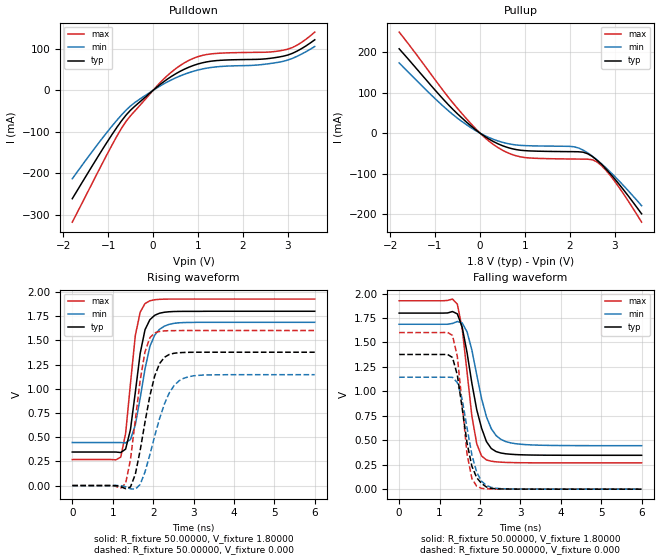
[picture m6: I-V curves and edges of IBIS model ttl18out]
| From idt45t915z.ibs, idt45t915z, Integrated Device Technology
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|   Model ttl18out
[Model]   ttl18out
Model_type   Output
Polarity   Non-Inverting
Vmeas =  0.90000V
C_comp   5.00000pF   5.00000pF   5.00000pF
[Temperature Range]   45.00000   0.14000k   -30.00000
[Voltage Range]   1.80000V   1.65000V   1.95000V
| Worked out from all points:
|   slope of the pulldown table from 0 to 0.27 V, typ, clamps not added: 11.6 ohm
|   slope of the pullup table from 0 to 0.27 V, typ, clamps not added: 14.1 ohm
|   rising waveform, R_fixture 50.00000, V_fixture 1.80000: 20-80 % time 293ps typ, 332ps min, 248ps max; typ from 0.346 V to 1.8 V
|   rising waveform, R_fixture 50.00000, V_fixture 0.000: 20-80 % time 385ps typ, 497ps min, 304ps max; typ from 0 V to 1.38 V
|   falling waveform, R_fixture 50.00000, V_fixture 1.80000: 20-80 % time 403ps typ, 417ps min, 289ps max; typ from 1.8 V to 0.346 V
|   falling waveform, R_fixture 50.00000, V_fixture 0.000: 20-80 % time 316ps typ, 322ps min, 240ps max; typ from 1.38 V to 0 V
[Pulldown]
| voltage   I(typ)   I(min)   I(max)
-1.8V     -261.1mA   -213mA     -317.7mA
-1V       -120.6mA   -97.41mA   -149mA
-600mV    -59.39mA   -47.53mA   -74.48mA
-400mV    -37.65mA   -28.88mA   -48.96mA
100mV     9.159mA    6.841mA    12.13mA
500mV     39.61mA    29.9mA     51.91mA
900mV     60mA       46.01mA    77.22mA
1.2V      68.62mA    53.53mA    86.39mA
2.5V      75.79mA    63.01mA    91.78mA
3V        85.05mA    72.93mA    99.21mA
3.3V      100.1mA    86.93mA    115mA
3.6V      121.7mA    105.6mA    140.3mA
[Pullup]
| voltage   I(typ)   I(min)   I(max)
-1.8V     208.2mA    173.4mA    249.5mA
-600mV    58.25mA    45.5mA     74.13mA
-100mV    8.512mA    6.375mA    11.27mA
200mV     -14.77mA   -10.9mA    -19.84mA
500mV     -31.12mA   -22.77mA   -42.22mA
900mV     -42.33mA   -30.33mA   -58.64mA
2.1V      -45.95mA   -33.9mA    -64.09mA
2.4V      -51.05mA   -48.94mA   -64.5mA
2.6V      -66.39mA   -65.62mA   -70.76mA
2.8V      -87.93mA   -85.25mA   -91.14mA
3V        -113.1mA   -106.9mA   -119mA
3.6V      -199.5mA   -179.5mA   -220.1mA
[Ramp]
| variable   typ   min   max
dV/dt_r   0.82620/0.39646n   0.68700/0.51978n   0.96060/0.30074n
dV/dt_f   0.87234/0.38849n   0.74820/0.41861n   0.99396/0.28717n
R_load = 50.00000
[Rising Waveform]
R_fixture = 50.00000
V_fixture = 1.80000
C_fixture = 0.000F
R_dut = 6.00000m
L_dut = 3.00000nH
C_dut = 0.20000pF
| time   V(typ)   V(min)   V(max)
0s        346.3mV    444.5mV    268.8mV
1.2ns     341.3mV    444.2mV    294mV
1.32ns    376.4mV    440.5mV    538.3mV
1.44ns    578.8mV    475.6mV    1.053V
1.56ns    963.4mV    626mV      1.55V
1.68ns    1.365V     902.9mV    1.79V
1.8ns     1.609V     1.205V     1.879V
2.04ns    1.758V     1.554V     1.919V
2.4ns     1.795V     1.665V     1.926V
6ns       1.8V       1.686V     1.926V
[Rising Waveform]
R_fixture = 50.00000
V_fixture = 0.000
C_fixture = 0.000F
R_dut = 6.00000m
L_dut = 3.00000nH
C_dut = 0.20000pF
| time   V(typ)   V(min)   V(max)
0s        0V         0V         0V
1.32ns    -32.39mV   -12.46mV   22.51mV
1.44ns    -14.55mV   -33.59mV   268.8mV
1.56ns    116mV      -37.24mV   676.2mV
1.68ns    363.8mV    11.28mV    1.087V
1.8ns     656.7mV    141.1mV    1.381V
2.04ns    1.133V     512.1mV    1.577V
2.4ns     1.354V     957mV      1.599V
2.76ns    1.375V     1.109V     1.601V
6ns       1.377V     1.145V     1.601V
[Falling Waveform]
R_fixture = 50.00000
V_fixture = 1.80000
C_fixture = 0.000F
R_dut = 6.00000m
L_dut = 3.00000nH
C_dut = 0.20000pF
| time   V(typ)   V(min)   V(max)
0s        1.8V       1.686V     1.926V
1.44ns    1.792V     1.714V     1.891V
1.56ns    1.655V     1.699V     1.643V
1.68ns    1.397V     1.609V     1.196V
1.8ns     1.081V     1.422V     745.9mV
1.92ns    812mV      1.168V     463.7mV
2.16ns    486.4mV    740mV      298.9mV
2.4ns     384.1mV    547.4mV    279.5mV
2.76ns    356.8mV    473.2mV    272.1mV
6ns       346.3mV    444.5mV    268.8mV
[Falling Waveform]
R_fixture = 50.00000
V_fixture = 0.000
C_fixture = 0.000F
R_dut = 6.00000m
L_dut = 3.00000nH
C_dut = 0.20000pF
| time   V(typ)   V(min)   V(max)
0s        1.377V     1.145V     1.601V
1.32ns    1.346V     1.143V     1.571V
1.44ns    1.166V     1.089V     1.355V
1.56ns    826.1mV    916.1mV    865.1mV
1.68ns    471.7mV    627mV      357.4mV
1.8ns     234.1mV    349.8mV    108.7mV
1.92ns    116.8mV    172.5mV    29.23mV
2.16ns    22.21mV    37.8mV     3.479mV
2.4ns     4.004mV    9.405mV    1.34mV
6ns       0V         3.198uV    0V
